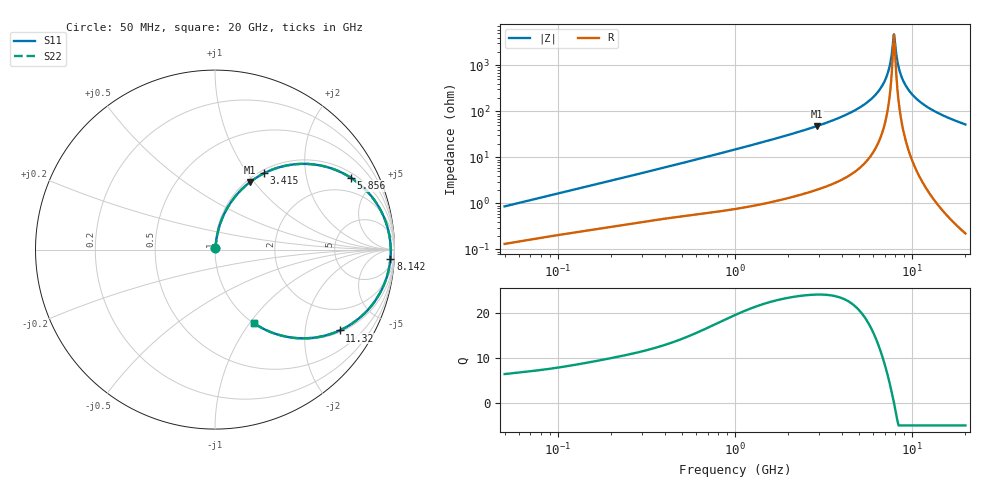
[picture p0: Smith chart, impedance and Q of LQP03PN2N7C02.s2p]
!Murata Part Number: LQP03PN2N7C02
!These Parameters are Measured in Series Mode Connection
!  o--[Z]--o
!Port1  Port2
!  o-------o
!Freq. Start=50[MHz] Stop=20[GHz], 401[Steps]
# Hz S RI R 50
!Freq.(Hz) S11(Real) S11(Imag) S21(Real) S21(Imag) S12(Real) S12(Imag) S22(Real) S22(Imag)
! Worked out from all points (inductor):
!   401 points, 50 MHz to 20 GHz, reference 50 ohm
!   read as one part in series: L = 2.67 nH near 51.52 MHz
!   highest Q = 24.2 at 2.896 GHz (marker M1), where L = 2.63 nH
!   self-resonance near 7.902 GHz
!   S11 on the Smith chart (normalised r, x): 50 MHz: 1.00, +0.02; 3.415 GHz: 1.05, +1.20; 5.856 GHz: 1.22, +3.67; 8.142 GHz: 14, -33; 11.32 GHz: 1.06, -3.04; 20 GHz: 1.00, -1.04
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5e7  0.00139 0.00851  0.9986 -0.00851  0.9986 -0.00851  0.00139 0.00851
1.364002e8  0.00294 0.0216  0.9971 -0.0216  0.9971 -0.0216  0.00294 0.0216
3.721004e8  0.00758 0.0556  0.9924 -0.0556  0.9924 -0.0556  0.00758 0.0556
1e9  0.0286 0.1432  0.9714 -0.1432  0.9714 -0.1432  0.0286 0.1432
1.793498e9  0.0789 0.2488  0.9211 -0.2488  0.9211 -0.2488  0.0789 0.2488
2.728004e9  0.1747 0.3596  0.8253 -0.3596  0.8253 -0.3596  0.1747 0.3596
2.896447e9  0.1965 0.3772  0.8035 -0.3772  0.8035 -0.3772  0.1965 0.3772
3.415248e9  0.2727 0.4251  0.7273 -0.4251  0.7273 -0.4251  0.2727 0.4251
4.677679e9  0.5104 0.4776  0.4896 -0.4776  0.4896 -0.4776  0.5104 0.4776
5.856089e9  0.7583 0.3994  0.2417 -0.3994  0.2417 -0.3994  0.7583 0.3994
6.802353e9  0.9115 0.2396  0.0885 -0.2396  0.0885 -0.2396  0.9115 0.2396
7.114996e9  0.944 0.1739  0.056 -0.1739  0.056 -0.1739  0.944 0.1739
7.442007e9  0.9666 0.1021  0.0334 -0.1021  0.0334 -0.1021  0.9666 0.1021
7.784049e9  0.978 0.0265  0.022 -0.0265  0.022 -0.0265  0.978 0.0265
8.020766e9  0.9789 -0.0249  0.0211 0.0249  0.0211 0.0249  0.9789 -0.0249
8.141811e9  0.9773 -0.0506  0.0227 0.0506  0.0227 0.0506  0.9773 -0.0506
8.516016e9  0.9646 -0.1263  0.0354 0.1263  0.0354 0.1263  0.9646 -0.1263
9.041845e9  0.9301 -0.2207  0.0699 0.2207  0.0699 0.2207  0.9301 -0.2207
9.892087e9  0.8491 -0.3388  0.1509 0.3388  0.1509 0.3388  0.8491 -0.3388
1.131968e10  0.694 -0.4506  0.306 0.4506  0.306 0.4506  0.694 -0.4506
1.504638e10  0.3959 -0.485  0.6041 0.485  0.6041 0.485  0.3959 -0.485
2e10  0.2148 -0.4085  0.7852 0.4085  0.7852 0.4085  0.2148 -0.4085
